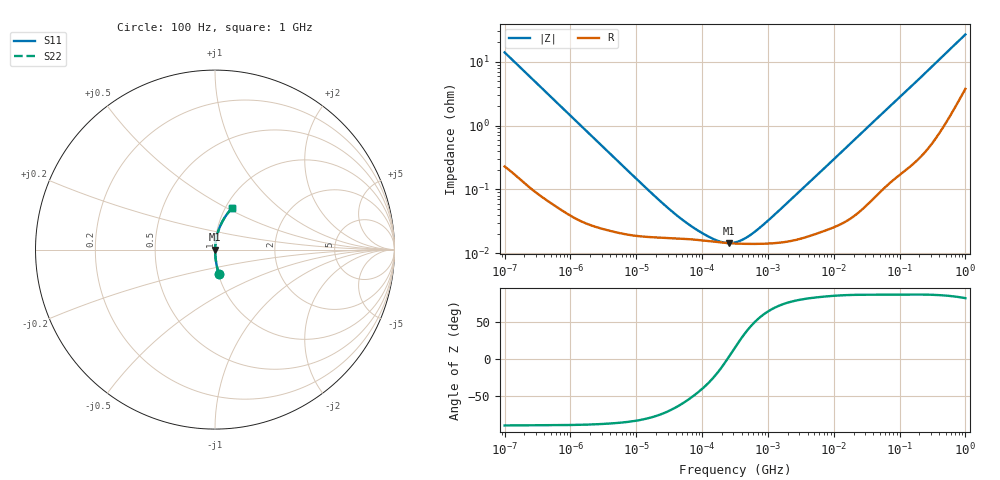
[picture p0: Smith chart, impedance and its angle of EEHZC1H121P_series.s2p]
!  *** S-Parameter ***
!  Copyright (C) Panasonic Industry
!  Conductive Polymer Hybrid Aluminum Electrolytic Capacitor
!  Parts No. EEHZC1H121P
!  Connection Mode : Series
!  1  o---||---o  2
!  GND o--------o GND
!  Conditions : Temperature = 20 degC , DC Bias = 0 V
! Frequency Range : 100Hz  -  1GHz  [ 401 Steps ]
# Hz S RI R 50
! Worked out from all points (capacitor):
!   401 points, 100 Hz to 1 GHz, reference 50 ohm
!   read as one part in series: C = 114 uF near 108.4 Hz
!   lowest |Z| = 14.5 mohm at 258.5 kHz (marker M1)
!   series resonance near 241.9 kHz, so ESL is about 3.8 nH
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100  0.0212 -0.1362  0.9788 0.1362  0.9788 0.1362  0.0212 -0.1362
108.3927  0.0184 -0.1262  0.9816 0.1262  0.9816 0.1262  0.0184 -0.1262
175.7924  0.00772 -0.0791  0.9923 0.0791  0.9923 0.0791  0.00772 -0.0791
309.0295  0.00295 -0.0455  0.997 0.0455  0.997 0.0455  0.00295 -0.0455
1487.647  0.000407 -0.00964  0.9996 0.00964  0.9996 0.00964  0.000407 -0.00964
22130.95  0.000177 -0.000662  0.9998 0.000662  0.9998 0.000662  0.000177 -0.000662
45708.82  0.000171 -0.000319  0.9998 0.000319  0.9998 0.000319  0.000171 -0.000319
90677.6  0.000161 -0.000151  0.9998 0.000151  0.9998 0.000151  0.000161 -0.000151
165958.7  0.00015 -5.43e-05  0.9998 5.43e-05  0.9998 5.43e-05  0.00015 -5.43e-05
211348.9  0.000147 -1.94e-05  0.9999 1.94e-05  0.9999 1.94e-05  0.000147 -1.94e-05
258523.5  0.000144 9.7e-06  0.9999 -9.7e-06  0.9999 -9.7e-06  0.000144 9.7e-06
316227.8  0.000143 3.99e-05  0.9999 -3.99e-05  0.9999 -3.99e-05  0.000143 3.99e-05
454464.5  0.000141 0.0001  0.9999 -0.0001  0.9999 -0.0001  0.000141 0.0001
707945.8  0.000141 0.000193  0.9999 -0.000193  0.9999 -0.000193  0.000141 0.000193
1244515  0.000145 0.000371  0.9999 -0.000371  0.9999 -0.000371  0.000145 0.000371
4704354  0.000195 0.00142  0.9998 -0.00142  0.9998 -0.00142  0.000195 0.00142
6.99842e7  0.00162 0.0195  0.9984 -0.0195  0.9984 -0.0195  0.00162 0.0195
1.631173e8  0.00447 0.0439  0.9955 -0.0439  0.9955 -0.0439  0.00447 0.0439
3.108136e8  0.012 0.082  0.988 -0.082  0.988 -0.082  0.012 0.082
5.922431e8  0.0375 0.1498  0.9625 -0.1498  0.9625 -0.1498  0.0375 0.1498
9.225714e8  0.0823 0.2165  0.9177 -0.2165  0.9177 -0.2165  0.0823 0.2165
1e9  0.0944 0.2298  0.9056 -0.2298  0.9056 -0.2298  0.0944 0.2298
